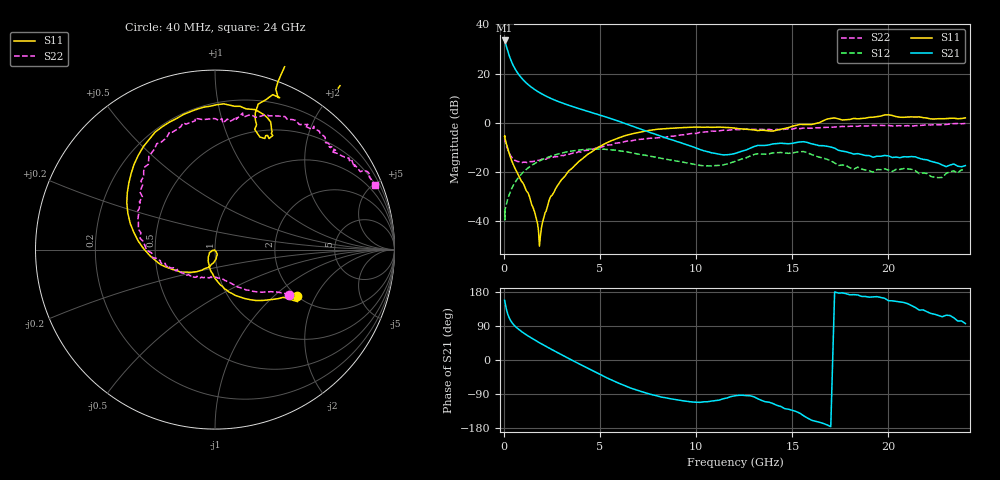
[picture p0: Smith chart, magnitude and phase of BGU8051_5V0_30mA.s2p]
! BGU8051_5V0_30mA
! Date/time Tue Jun 16 10:58:09 2015
! VAR V_out= 5.0000
! VAR I_out= 29.9650
! VAR V_in= 3.7170
! VAR I_in= 0.3871
# MHz S MA R 50
!  Freq-MHz  S11-mag  S11-arg  S21-mag  S21-arg  S12-mag  S12-arg  S22-mag  S22-arg
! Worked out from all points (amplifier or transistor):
!   187 points, 40 MHz to 24 GHz, reference 50 ohm
!   highest |S21| = 33.5 dB at 40 MHz (marker M1)
!   |S21| within 3 dB of that: start of sweep to 156.3 MHz
!   unconditionally stable (mu >= 1): 626.6 MHz to 14.08 GHz
!   at 750 MHz: K = 1.01, MAG = 20.6 dB, |S12| = -22.5 dB
!   at 5.4 GHz: K = 1.21, MAG = 3.7 dB, |S12| = -10.9 dB
!   at 24 GHz: K = -0.82, MSG = 1.0 dB, |S12| = -19.5 dB
!   lowest NFmin = 0.30 dB at 400 MHz
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40  0.5269 -29.3  47.24 157.6  0.01583 33.5  0.4856 -31.3
50  0.5442 -32.2  45.91 155.6  0.01456 -22.1  0.4682 -31.7
60  0.468 -34.7  45.12 152.5  0.01044 36.7  0.4333 -33.5
80  0.4491 -37.4  42.13 147.1  0.01785 35.8  0.4026 -35.8
120  0.3901 -46.5  37.49 137.0  0.02082 40.6  0.3537 -42.1
180  0.3167 -59.1  31.05 125.0  0.02556 48.3  0.2982 -49.6
240  0.2623 -68.8  25.97 115.9  0.03072 52.2  0.2591 -55.7
300  0.2236 -76.5  22.07 109.0  0.03588 54.5  0.2312 -60.3
360  0.1888 -83.2  19.05 103.5  0.04068 56.5  0.2095 -64.1
440  0.1555 -90.8  16.05 97.6  0.04786 57.9  0.1917 -69.0
550  0.1244 -100.1  13.16 91.0  0.0576 58.4  0.1733 -73.9
750  0.08744 -112.6  9.857 81.8  0.0754 57.5  0.1609 -82.0
950  0.06196 -127.4  7.867 74.0  0.09281 55.2  0.1539 -88.8
1600  0.0152 -161.1  4.739 53.0  0.1469 43.8  0.1639 -109.3
1850  0.003047 -124.1  4.105 45.6  0.166 38.8  0.1721 -116.5
2600  0.0379 -76.3  2.931 24.7  0.217 23.0  0.2002 -132.7
4100  0.1852 -136.9  1.83 -15.1  0.2819 -9.9  0.2559 -156.3
8200  0.7458 112.9  0.525 -98.0  0.188 -77.1  0.4981 147.8
12200  0.7551 65.5  0.2486 -93.2  0.1725 -71.8  0.7176 103.0
16200  0.9551 69.2  0.3566 -161.7  0.2097 -150.7  0.7868 70.9
20200  1.398 34.5  0.1952 156.1  0.1012 -160.8  0.857 44.0
24000  1.252 21.1  0.1334 96.2  0.1058 -175.7  0.9627 21.8
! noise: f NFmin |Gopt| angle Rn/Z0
400  0.302  0.1998  29.1  0.0515
550  0.3158  0.1687  37.72  0.0515
950  0.3632  0.116  71.04  0.0511
1250  0.4091  0.1084  101.7  0.0504
1600  0.4736  0.1234  130.4  0.0497
1900  0.5383  0.1433  147.2  0.0495
2250  0.6249  0.167  161.7  0.0501
2600  0.7234  0.1892  173.3  0.052
3300  0.9561  0.232  192.4  0.0612
4000  1.236  0.2793  207.3  0.0805
